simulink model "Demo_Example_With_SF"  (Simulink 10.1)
settings: Solver=FixedStepDiscrete  StartTime=0.0  StopTime=100  FixedStep=1  RelTol=1e-3
undefined symbols (not defined in the file or in its folder): e_NotTripped, e_Tripped, k_Hys, k_Setpoint

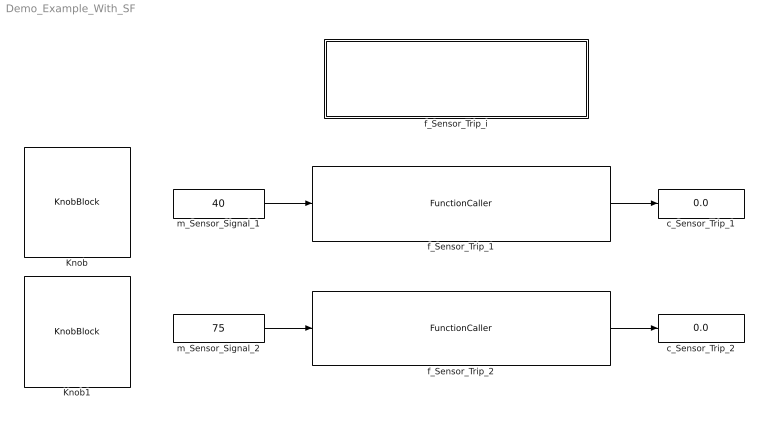
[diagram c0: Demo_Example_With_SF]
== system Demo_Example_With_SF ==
  Knob : KnobBlock
  Knob1 : KnobBlock
  c_Sensor_Trip_1 : Display
  c_Sensor_Trip_2 : Display
  f_Sensor_Trip_1 : FunctionCaller  FunctionPrototype=c_Sensor_Trip_i = f_Sensor_Trip_i(m_Sensor_Signal_i)  InputArgumentSpecifications=int16(1)  OutputArgumentSpecifications=boolean(1)
  f_Sensor_Trip_2 : FunctionCaller  FunctionPrototype=c_Sensor_Trip_i = f_Sensor_Trip_i(m_Sensor_Signal_i)  InputArgumentSpecifications=int16(1)  OutputArgumentSpecifications=boolean(1)
  f_Sensor_Trip_i : Subsystem
  m_Sensor_Signal_1 : Constant  Value=40  OutDataTypeStr=int16
  m_Sensor_Signal_2 : Constant  Value=75  OutDataTypeStr=int16
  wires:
  f_Sensor_Trip_1/1 -> c_Sensor_Trip_1/1
  f_Sensor_Trip_2/1 -> c_Sensor_Trip_2/1
  m_Sensor_Signal_1/1 -> f_Sensor_Trip_1/1
  m_Sensor_Signal_2/1 -> f_Sensor_Trip_2/1

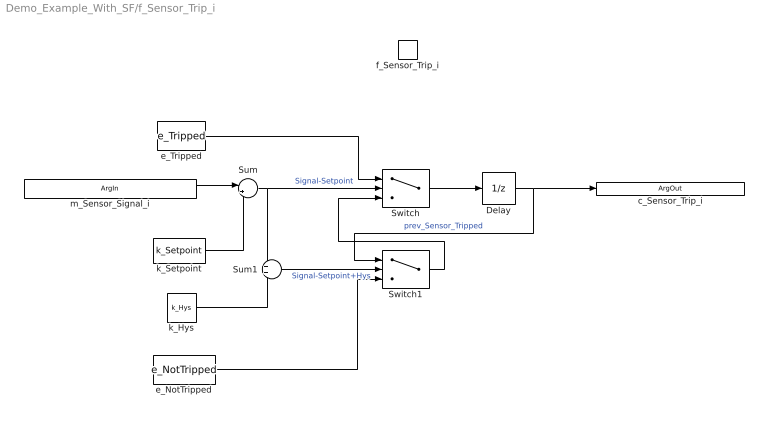
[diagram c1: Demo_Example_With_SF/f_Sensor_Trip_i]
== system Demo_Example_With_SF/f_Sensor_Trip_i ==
  f_Sensor_Trip_i : TriggerPort  TriggerType=function-call  IsSimulinkFunction=on  FunctionName=f_Sensor_Trip_i  FunctionVisibility=scoped  VariantControl=Variant  PortDimensions=1
  Delay : UnitDelay  SampleTime=-1  HasFrameUpgradeWarning=on
  Sum : Sum  Inputs=|+-  AccumDataTypeStr=int16
  Sum1 : Sum  AccumDataTypeStr=int16
  Switch : Switch  OutDataTypeStr=boolean
  Switch1 : Switch  OutDataTypeStr=boolean
  e_NotTripped : Constant  Value=e_NotTripped  OutDataTypeStr=boolean
  e_Tripped : Constant  Value=e_Tripped  OutDataTypeStr=boolean
  k_Hys : Constant  Value=k_Hys  OutDataTypeStr=int16
  k_Setpoint : Constant  Value=k_Setpoint  OutDataTypeStr=int16
  m_Sensor_Signal_i : ArgIn  OutDataTypeStr=int16  ArgumentName=m_Sensor_Signal_i
  c_Sensor_Trip_i : ArgOut  OutDataTypeStr=boolean  ArgumentName=c_Sensor_Trip_i
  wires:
  m_Sensor_Signal_i/1 -> Sum/1
  Sum/1 -> Switch/2, Sum1/1  "Signal-Setpoint"
  e_Tripped/1 -> Switch/1
  Switch/1 -> Delay/1
  Delay/1 -> Switch1/1, c_Sensor_Trip_i/1  "prev_Sensor_Tripped"
  Switch1/1 -> Switch/3
  k_Hys/1 -> Sum1/2
  Sum1/1 -> Switch1/2  "Signal-Setpoint+Hys"
  e_NotTripped/1 -> Switch1/3
  k_Setpoint/1 -> Sum/2
